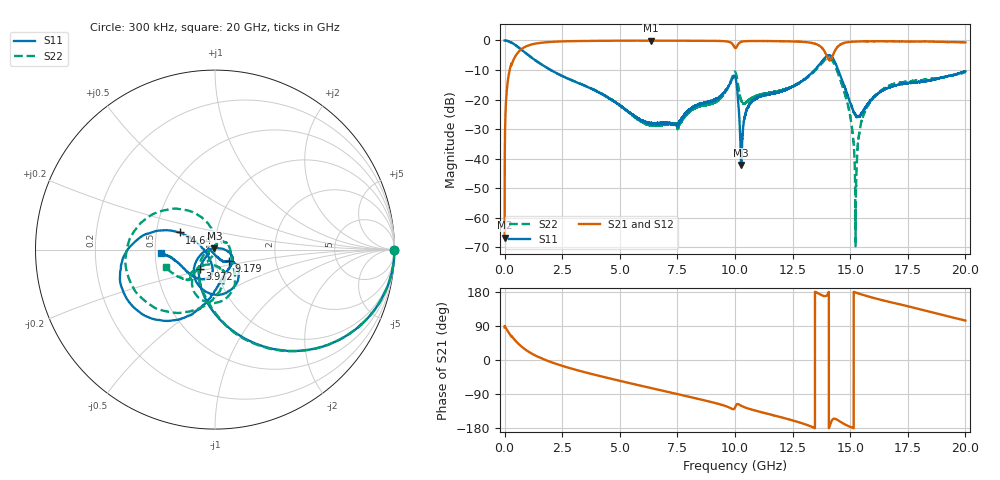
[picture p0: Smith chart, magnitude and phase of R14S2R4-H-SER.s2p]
!{R14S2R4}
!Johanson Technology Inc.
!www.johansontechnology.com
!Test Board Conditions:
!Substrate Type  RO4350B
!Substrate Thickness  20 mil
!Substrate Dk  3.66
!TL Type: GCPW
!TL Trace Width  36 mil
!TL Gap  12 mil
!Electrode orientation  Horizontal
!DUT TOPOLOGY	SERIES
!Mounting Pad LxW  26x36 mil
! Created Wed Nov 25 17:33:21 2020
! 2 Port Network Data from SP1.SP block
! freq  magS11  angS11  magS21  angS21  magS12  angS12  magS22  angS22
# khz S ma R 50
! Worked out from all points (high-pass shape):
!   20001 points, 300 kHz to 20 GHz, reference 50 ohm
!   highest |S21| = -0.05 dB at 6.35 GHz (marker M1); lowest = -66.8 dB at 300 kHz (marker M2)
!   |S21| within 3 dB of the highest: 714.2 MHz to 13.84 GHz (13.12 GHz wide, 180 % of centre); 14.37 GHz to end of sweep
!   lowest |S11| = -42.1 dB at 10.26 GHz (marker M3), VSWR 1.02, Z = 49.6 + j0.695 ohm
!   |S11| at or under -10 dB: 2.005 GHz to 13.46 GHz (11.45 GHz wide, 148 % of centre); 14.48 GHz to end of sweep
!   |S22| runs from -69.6 to 0.0 dB; largest |S21 - S12| = 0.02
!   S11 on the Smith chart (normalised r, x): 300 kHz: open; 3.972 GHz: 0.82, -0.19; 9.179 GHz: 1.16, -0.15; 14.64 GHz: 0.66, +0.13; 20 GHz: 0.54, -0.02
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300  0.9987 -0.2  0.0004596 86.2  0.0004699 87.0  0.9991 -0.3
129300  0.9803 -12.8  0.1925 77.0  0.1931 77.0  0.9808 -12.8
465300  0.8384 -38.3  0.5398 51.4  0.5408 51.5  0.8377 -38.3
1457300  0.4274 -81.6  0.8993 8.1  0.8999 8.1  0.4279 -81.8
3334300  0.1806 -119.5  0.978 -29.9  0.9784 -29.9  0.1825 -119.1
3972300  0.1393 -127.7  0.9846 -39.9  0.9849 -39.9  0.1409 -130.3
6350300  0.04022 -153.7  0.9939 -74.0  0.9919 -74.0  0.03696 -174.6
6667300  0.03938 -159.4  0.9915 -78.4  0.9915 -78.3  0.03681 -174.3
9179300  0.1015 -39.1  0.9821 -114.1  0.984 -114.2  0.09248 -16.0
1.00003e7  0.2451 -97.5  0.7451 -125.7  0.7461 -125.6  0.2976 -96.1
1.02603e7  0.007856 117.1  0.9447 -120.5  0.9461 -120.5  0.09967 -121.5
1.07983e7  0.09794 -18.6  0.9781 -132.1  0.9768 -132.1  0.1087 -74.5
1.33343e7  0.2824 -97.7  0.907 -176.3  0.9099 -176.4  0.2727 -91.7
1.38333e7  0.4739 -123.1  0.7056 169.4  0.709 168.8  0.4383 -128.3
1.41053e7  0.5615 -156.9  0.4599 -174.9  0.4603 -175.5  0.5042 -172.0
1.46383e7  0.2194 154.2  0.88 -165.4  0.8773 -165.3  0.1806 110.0
1.49963e7  0.08919 162.8  0.9466 -176.3  0.9452 -176.3  0.05279 86.6
1.52423e7  0.0536 -163.7  0.9597 178.0  0.9599 178.0  0.001786 -110.9
1.54213e7  0.05264 -132.9  0.966 174.4  0.9657 174.3  0.03112 -113.3
1.56293e7  0.07117 -109.5  0.9685 170.4  0.9689 170.5  0.06165 -118.1
1.66673e7  0.1585 -101.9  0.9677 153.8  0.9635 153.7  0.1704 -135.2
2e7  0.3004 -176.4  0.9272 104.0  0.9246 104.2  0.2901 -160.3
